//05.04.99
//Umstrukturierung, Aufruf FB2 mit Multiinstanz-DB
//Lesen von numMagPlaceParam bei Neustart da Änderung Anzahl Par. in SW 5 (8)
//DB99 und DB100 entfallen da Aufruf FB2 mit Multiiinstanz-DB
//neue Fkt: TNr_write=1, Vorgabe TNummer in TNr von extern
//

FUNCTION_BLOCK FB 93
TITLE = ZU_PUT
VERSION : 2.0

VAR_INPUT
    Req:	Bool; // Start Zustände schreiben
    PutWkz:     Bool; // Werkzeugzustand schreiben
    MagNr:	Int; // Magazin-Nr. Daten schreiben
    LocNr:	Int; // Platz-Nr. Daten schreiben
END_VAR

VAR_OUTPUT
    Done:	Bool; // Schreiben beendet
    Error:	Bool; // Fehler
    State:	Word; // Fehler-Nummer
END_VAR

VAR
    TOANr: Byte:=b#16#1; // TOA-Bereich
    TNr_write: Bool:=False; // T-Nummer von Anwender versorgt
    numMagPlaceParams: Word; // Anzahl Parameter eines Magzinplatzes
    numPlacePar_read: Bool; //Variable nummagplaceparams lesen nach Neustart
    numPlacePar_Error: Bool; // Fehler bei Variable nummagplaceparams lesen
    numPlacePar_ok: Bool; // Variable numMagPlaceParams gelesen ohne Fehler
    Activ: Bool; // Baustein aktiv
    Schrittregister : BYTE ;
    StateFB2_Gesp: Word; // Ausgang State FB2 gespeichert
    StateFB3_Gesp: Word; // Ausgang State FB3 gespeichert
    ColumnMagNr: Word; // Spaltenadresse für Magazin-Nummer
    LocLineTNr: Word; // Zeilenadresse für T-Nummer
    LocLinePlz: Word; // Zeilenadresse für Platzzustand
    Reserve: ARRAY  [0 .. 2 ] OF Int;
    TNr: Int; // logische T-Nummer
    Loc_Zu:	Int; // Platzzustand aktuell
    Loc_ZuPut: Int; // Platzzustand schreiben
    WZStatus: Int; // Werkzeugstatus
    GET_FB2: FB 2;
    PUT_FB3: FB3;
END_VAR

VAR_TEMP
    Error_FB2: Bool; // Error FB2
    NDR_FB2: Bool; // Auftrag beendet FB2
    Error_FB3: Bool; // Error FB3
    Done_FB3: Bool; // Auftrag beendet FB3
    State_FB2: Word; // Fehler-Nr. FB2
    State_FB3: Word; // Fehler-Nr. FB3
    LocLine1: Word; // Zeilenadresse Addr1
END_VAR


Begin
     UN   DB8.DBX45.0;
     SPB  ANF1;		// Neustart ? Nein ->
     CALL #GET_FB2 (
     Req:= FALSE);
     SET;
     R    numPlacePar_Error;
     S    numPlacePar_read;
     R    numPlacePar_ok;
     SPA  LOEP;
ANF1:UN   numPlacePar_read;
     SPB  ANF2;
     call #GET_FB2 ( // -- Anzahl Parameter eines Magazinplatz lesen --
     Req:=TRUE, // Variable lesen
     NumVar:= 1, // Anzahl der zu lesenden Variablen
     Addr1:=WZV_VAR.N_Y_numMagPlaceParams_27, // Variable numMagPlaceParams
     Error:=#Error_FB2, // NC_VAR lesen beendet mit Fehler
     NDR:=#NDR_FB2, // NC_VAR lesen beendet ohne Fehler
     State:=#State_FB2, // Fehler-Nummer bei Error = 1
     RD1:=numMagPlaceParams); // Wert in numMagPlaceParams
     UN    #NDR_FB2; // Lesen beendet ohne Fehler
     UN    #Error_FB2; // Lesen beendet mit Fehler
     SPB   ENDE; // Lesen beendet ? Nein ->
     call #GET_FB2 ( // FB2 freigeben
     Req:=False);
     UN    #Error_FB2;
     R     numPlacePar_read;
     S     numPlacePar_ok;
     SPB   ENDE; // Lesen beendet mit Fehler ? Nein ->
     L     6;
     L     #State_FB2;
     ==I;
     SPB   ENDE; // FIFO voll -> Lesen wiederholen
     S     numPlacePar_Error;
     R     numPlacePar_read;
     T     StateFB2_Gesp; // Fehlernummer speichern
     SPA   ENDE;
ANF2:U   Req;
     SPB ANF;
LOEP:R    Done; // Ausgangsparameter Done nur 1 PLC-Zyklus
     R    Error; // Ausgangsparameter Error nur 1 PLC-Zyklus
     R    Activ;
     L    0;
     T    State; // Fehler-Nr. = 0
     SPA  ENDE;
ANF: U    Activ;
     SPB  SPRG; // Baustein aktiv ? Ja ->
     U   numPlacePar_Error;
     ON  numPlacePar_ok;
     L	7;
     SPB  FEHL; // Fehler bei Variable numMagPlaceParams lesen ->
     S    Activ; // Hilfsvariable vorbesetzen
     R    Done;
     R    Error;
     L    0;
     T    State; // Fehler-Nr. = 0
     UN   PutWkz;
     SPB  SR; // MagPlatzdaten schreiben ? ->
     L    1;
SR:  T    Schrittregister;
     L    MagNr; //
     T    ColumnMagNr; // Spalte Addr = Magazin-Nummer
     L    LocNr; // Platz-Nr. Zwischenspeicher
     +    -1;
     L    numMagPlaceParams; // Anzahl Parameter pro MagPlatz
     *I; // (PlatzNr.-1)*numMagPlaceParams+Parameter-Nr.
     +    3;
     T    LocLineTNr; // Zeilenadresse für TNr
     +    2;
     T    LocLinePlz; // Zeilenadresse für Platzzustand
SPRG:L    Schrittregister;
     SPL  FEHS; // Sprungverteiler
     SPA  SR1; // Magazinplatzdaten schreiben
     SPA  SR2; // Magazinplatzdaten lesen
     SPA  SR3; // Werkzeugstatus schreiben
FEHS:L 6;
     SPA  FEHL;
SR1: call PUT_FB3( // ----Schritt 1: Magazinplatzdaten schreiben
     Req:=TRUE, // Variable Magazinplatz-Daten schreiben
     NumVar:=1,
     Addr1:=WZV_VAR.T0_TP_placeData0_0, // Platzzustand
     Unit1:=TOANr, // Bereich = TOA 1
     Column1:=#ColumnMagNr, //Spaltenadresse Magazinnummer
     Line1:=#LocLinePlz, // Zeilenadresse Platzzustand
     Error:=Error_FB3,
     Done:=Done_FB3,
     State:=State_FB3,
     SD1:=Loc_ZuPut); // Magazinplatzzustand
     UN    #Done_FB3; // Lesen beendet ohne Fehler
     UN    #Error_FB3; // Lesen beendet mit Fehler
     SPB   ENDE; // Lesen beendet ? Nein ->
     call #PUT_FB3 ( // FB2 freigeben
     Req:=False);
     UN    #Error_FB3;
     SPB   DONE; // Lesen beendet mit Fehler ? Nein ->
     L     6;
     L     #State_FB3;
     ==I;
     SPB   ENDE;
     T     StateFB3_Gesp; // Fehlernummer speichern
     L     4; // Fehler-Nummer FB 93 = 4
     SPA   FEHL;
SR2: U     TNr_write; // -- Magazinplatzdaten lesen --
     SPB   QFE1; // T-Nr extern ? ->
     call #GET_FB2 (
     Req:=TRUE, // Variable lesen
     NumVar:= 2, // Anzahl der zu lesenden Variablen
     Addr1:=WZV_VAR.T0_TP_placeData0_0, // T-Nummer von WZ in Zwischenspeicher
     Unit1:=TOANr, // Bereich = TOA 1
     Column1:=#ColumnMagNr, // Spaltenadresse
     Line1:=#LocLineTNr, // Zeilenadresse
     Addr2:=WZV_VAR.T0_TP_placeData0_0, // T-Nummer von WZ in Zwischenspeicher
     Unit2:=TOANr, // Bereich = TOA 1
     Column2:=#ColumnMagNr, // Spaltenadresse
     Line2:=#LocLinePlz, // Zeilenadresse
     Error:=#Error_FB2, // NC_VAR lesen beendet mit Fehler
     NDR:=#NDR_FB2, // NC_VAR lesen beendet ohne Fehler
     State:=#State_FB2, // Fehler-Nummer bei Error = 1
     RD1:=TNr, // Zielbereich für T-Nummer
     RD2:=Loc_Zu); // Zielbereich für  Platzzustand
     UN    #NDR_FB2; // Lesen beendet ohne Fehler
     UN    #Error_FB2; // Lesen beendet mit Fehler
     SPB   ENDE; // Lesen beendet ? Nein ->
     call #GET_FB2 ( // FB2 freigeben
     Req:=False);
     UN    #Error_FB2;
     SPB   QFE1; // Lesen beendet mit Fehler ? Nein ->
     L     6;
     L     #State_FB2;
     ==I;
     SPB   ENDE;
     T     StateFB2_Gesp; // Fehlernummer speichern
     L     1; // Fehler-Nummer FB 91 = 1
     SPA   FEHL;
QFE1:L     TNr;	// logische T-Nummer von WZ in Zwischenspeicher
     L     0;
     ==I;
     L     2;
     SPB   FEHL; // T-Nr. in Zwischensp. = 0 ? -> Fehler
     L     2;
     T     Schrittregister;
SR3: L     TNr; // logische T-Nr. = Zeilenadresse          L     TNr; // logische T-Nr. = Zeilenadresse
     T     #LocLine1;
     call PUT_FB3(
     Req:=TRUE, // Variable WZ-Daten schreiben
     NumVar:=1,
     Addr1:=WZV_VAR.T0_TD_toolState0_0, // Größe nach links in Halbplätze
     Unit1:=TOANr, // Bereich = TOA 1
     Column1:=w#16#0008, // Spalte = WZ-Status
     Line1:=#LocLine1, // Zeilenadresse= TNr
     Error:=Error_FB3,
     Done:=Done_FB3,
     State:=State_FB3,
     SD1:=WZStatus); // WZ-Status
     UN    #Done_FB3; // Lesen beendet ohne Fehler
     UN    #Error_FB3; // Lesen beendet mit Fehler
     SPB   ENDE; // Lesen beendet ? Nein ->
     call #PUT_FB3 ( // FB2 freigeben
     Req:=False);
     UN    #Error_FB3;
     SPB   DONE; // Lesen beendet mit Fehler ? Nein ->
     L     6;
     L     #State_FB3;
     ==I;
     SPB   ENDE;
     T     StateFB3_Gesp; // Fehlernummer speichern
     L     3; // Fehler-Nummer FB 93 = 3
     SPA   FEHL;
DONE:S     Done;
     SPA   SR0;
FEHL:T     State; // Fehler-Nummer FB92 ausgeben
     S     Error;
SR0: R     Activ;
     L     0;
     T     Schrittregister; // Schrittregister auf Anfang
ENDE:NOP   0
END_FUNCTION_BLOCK

DATA_BLOCK db 93

        VERSION: 2.0

fb 93
Begin
END_DATA_BLOCK

